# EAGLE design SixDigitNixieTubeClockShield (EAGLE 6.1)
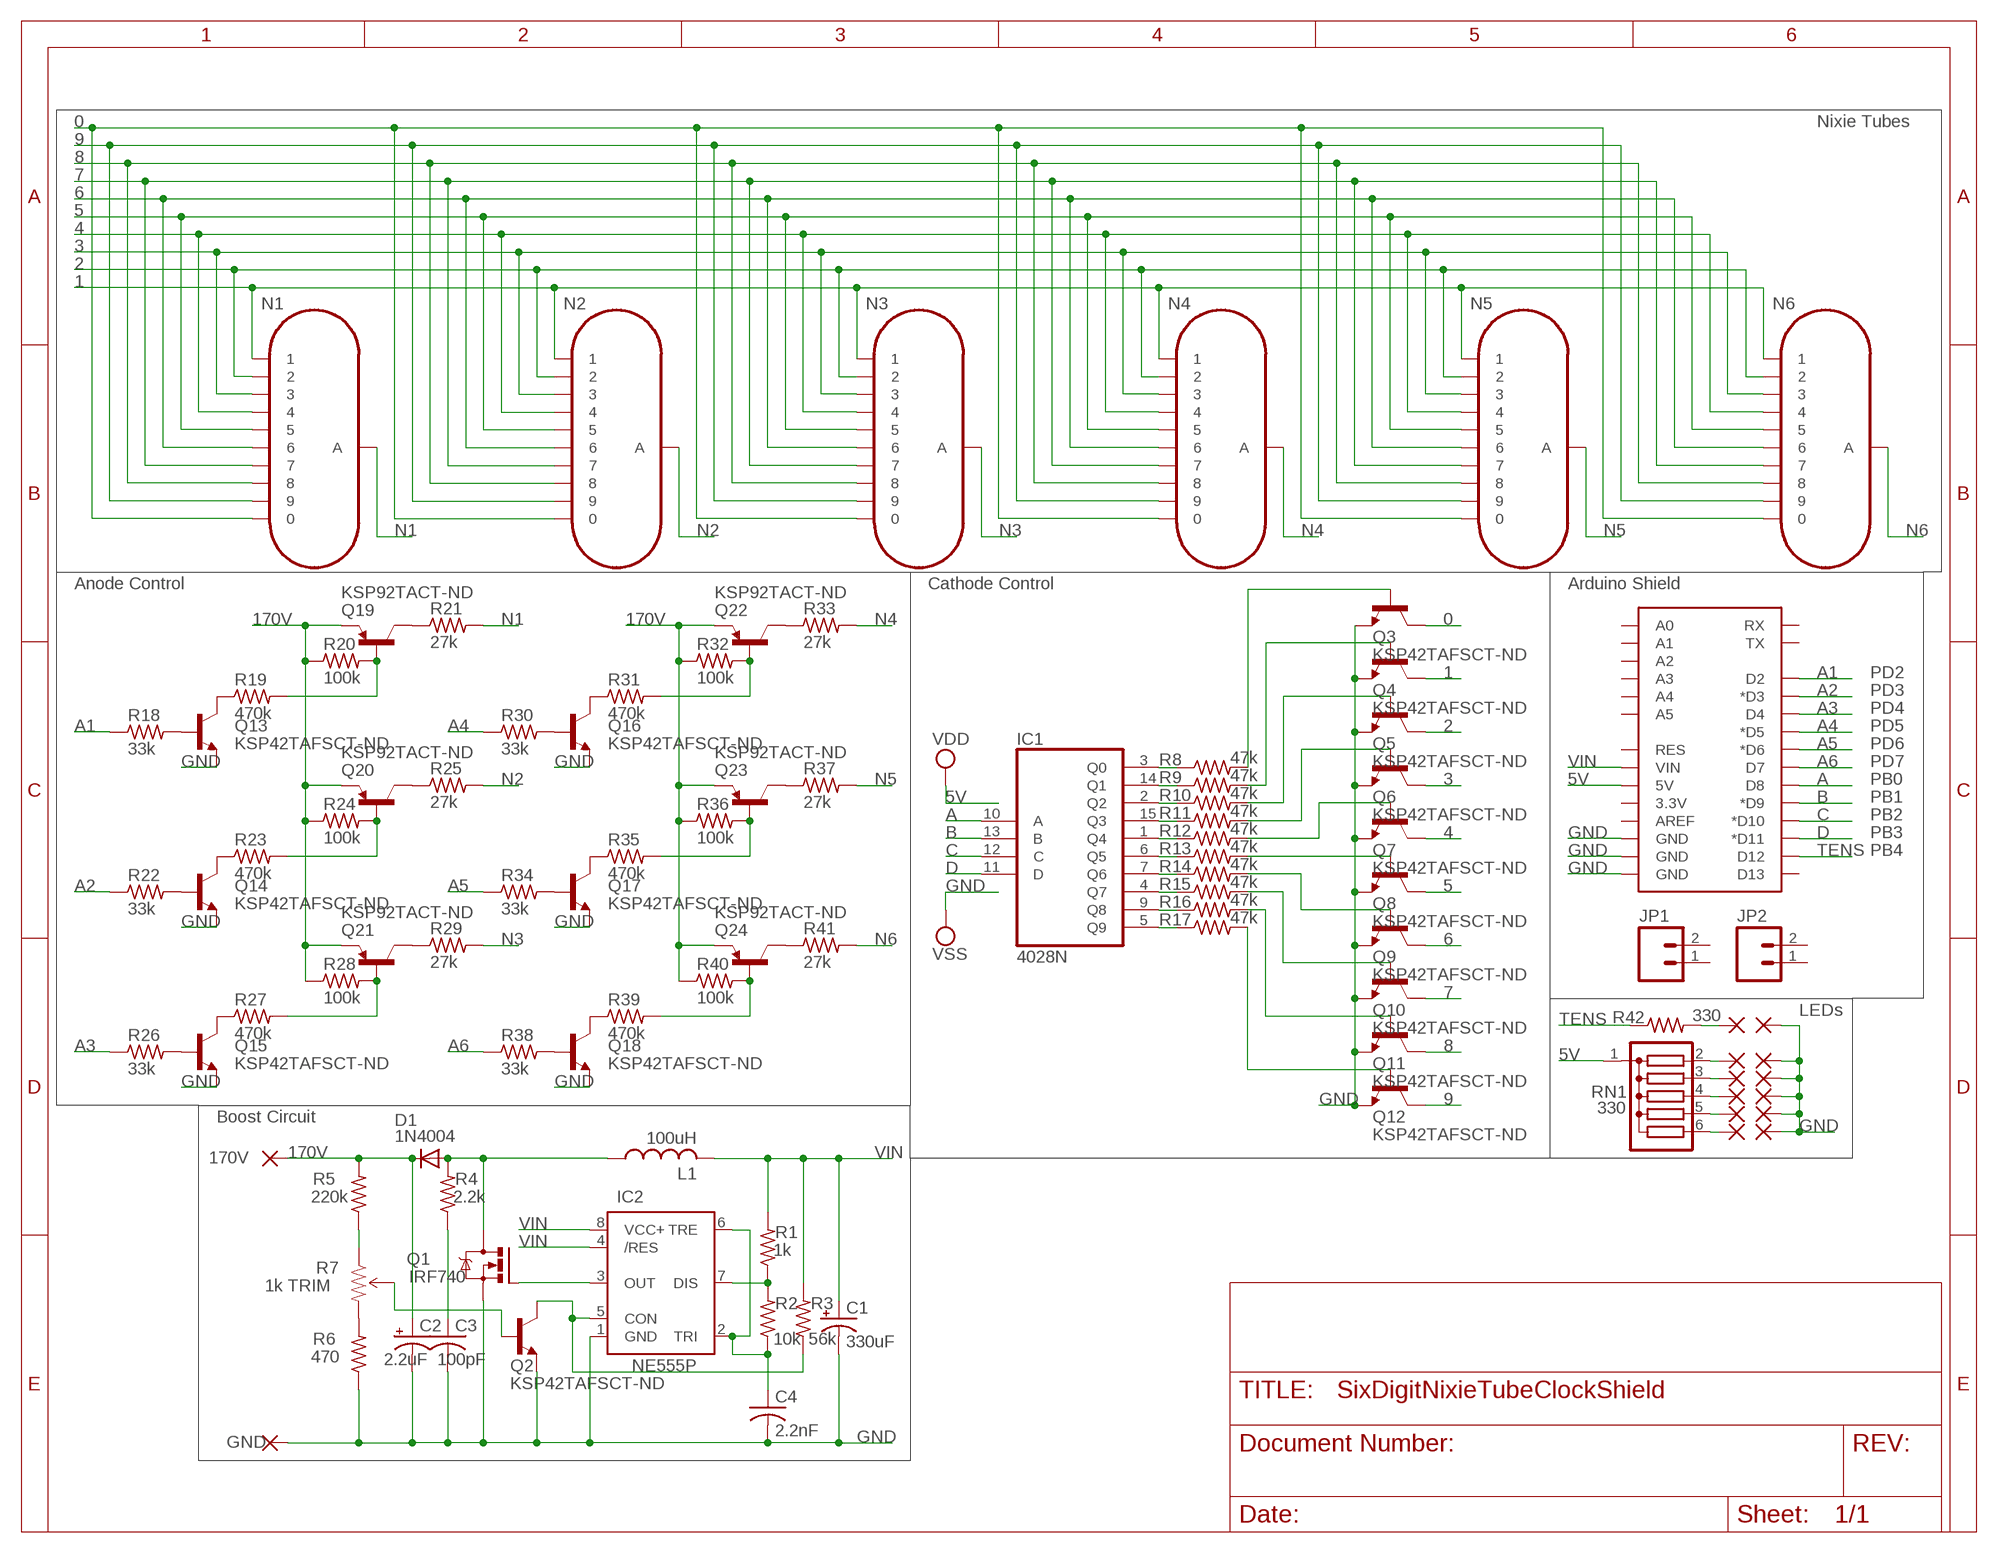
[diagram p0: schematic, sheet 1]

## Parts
C1  330uF  CPOL-USE2,5-6E  [E2,5-6E]
C2  2.2uF  CPOL-USE2,5-6E  [E2,5-6E]
C3  100pF  C-US050-025X075  [C050-025X075]
C4  2.2nF  C-US025-025X050  [C025-025X050]
D1  1N4004  [DO41-10]
IC1  4028N  [DIL16]
IC2  NE555P  [DIL-08]
JP1  M02PTH  [1X02]
JP2  M02PTH  [1X02]
L1  100uH  L-US6000-XXX-RC  [6000-XXXX-RC]
N1  IN-17  [IN-17]
N2  IN-17  [IN-17]
N3  IN-17  [IN-17]
N4  IN-17  [IN-17]
N5  IN-17  [IN-17]
N6  IN-17  [IN-17]
PAD1  1,6/0,8  [1,6/0,8]
PAD2  1,6/0,8  [1,6/0,8]
PAD3  1,6/0,8  [1,6/0,8]
PAD4  1,6/0,8  [1,6/0,8]
PAD5  1,6/0,8  [1,6/0,8]
PAD6  1,6/0,8  [1,6/0,8]
PAD7  1,6/0,8  [1,6/0,8]
PAD8  1,6/0,8  [1,6/0,8]
PAD9  1,6/0,8  [1,6/0,8]
PAD10  1,6/0,8  [1,6/0,8]
PAD11  1,6/0,8  [1,6/0,8]
PAD12  1,6/0,8  [1,6/0,8]
PAD13  GND  1,6/0,8  [1,6/0,8]
PAD14  170V  1,6/0,8  [1,6/0,8]
Q1  IRF740  [TO220BV]
Q2  KSP42TAFSCT-ND  TRANSISTOR_NPNTO-92-AMMO  [TO-92-AMMO]
Q3  KSP42TAFSCT-ND  TRANSISTOR_NPNTO-92-AMMO  [TO-92-AMMO]
Q4  KSP42TAFSCT-ND  TRANSISTOR_NPNTO-92-AMMO  [TO-92-AMMO]
Q5  KSP42TAFSCT-ND  TRANSISTOR_NPNTO-92-AMMO  [TO-92-AMMO]
Q6  KSP42TAFSCT-ND  TRANSISTOR_NPNTO-92-AMMO  [TO-92-AMMO]
Q7  KSP42TAFSCT-ND  TRANSISTOR_NPNTO-92-AMMO  [TO-92-AMMO]
Q8  KSP42TAFSCT-ND  TRANSISTOR_NPNTO-92-AMMO  [TO-92-AMMO]
Q9  KSP42TAFSCT-ND  TRANSISTOR_NPNTO-92-AMMO  [TO-92-AMMO]
Q10  KSP42TAFSCT-ND  TRANSISTOR_NPNTO-92-AMMO  [TO-92-AMMO]
Q11  KSP42TAFSCT-ND  TRANSISTOR_NPNTO-92-AMMO  [TO-92-AMMO]
Q12  KSP42TAFSCT-ND  TRANSISTOR_NPNTO-92-AMMO  [TO-92-AMMO]
Q13  KSP42TAFSCT-ND  TRANSISTOR_NPNTO-92-AMMO  [TO-92-AMMO]
Q14  KSP42TAFSCT-ND  TRANSISTOR_NPNTO-92-AMMO  [TO-92-AMMO]
Q15  KSP42TAFSCT-ND  TRANSISTOR_NPNTO-92-AMMO  [TO-92-AMMO]
Q16  KSP42TAFSCT-ND  TRANSISTOR_NPNTO-92-AMMO  [TO-92-AMMO]
Q17  KSP42TAFSCT-ND  TRANSISTOR_NPNTO-92-AMMO  [TO-92-AMMO]
Q18  KSP42TAFSCT-ND  TRANSISTOR_NPNTO-92-AMMO  [TO-92-AMMO]
Q19  KSP92TACT-ND  TRANSISTOR_PNP  [TO-92-AMMO]
Q20  KSP92TACT-ND  TRANSISTOR_PNP  [TO-92-AMMO]
Q21  KSP92TACT-ND  TRANSISTOR_PNP  [TO-92-AMMO]
Q22  KSP92TACT-ND  TRANSISTOR_PNP  [TO-92-AMMO]
Q23  KSP92TACT-ND  TRANSISTOR_PNP  [TO-92-AMMO]
Q24  KSP92TACT-ND  TRANSISTOR_PNP  [TO-92-AMMO]
R1  1k  R-US_0204/5  [0204/5]
R2  10k  R-US_0204/5  [0204/5]
R3  56k  R-US_0204/5  [0204/5]
R4  2.2k  R-US_0204/5  [0204/5]
R5  220k  R-US_0204/5  [0204/5]
R6  470  R-US_0204/5  [0204/5]
R7  1k TRIM  TRIMPOTPTH  [TRIM_POT_PTH]
R8  47k  R-US_0204/5  [0204/5]
R9  47k  R-US_0204/5  [0204/5]
R10  47k  R-US_0204/5  [0204/5]
R11  47k  R-US_0204/5  [0204/5]
R12  47k  R-US_0204/5  [0204/5]
R13  47k  R-US_0204/5  [0204/5]
R14  47k  R-US_0204/5  [0204/5]
R15  47k  R-US_0204/5  [0204/5]
R16  47k  R-US_0204/5  [0204/5]
R17  47k  R-US_0204/5  [0204/5]
R18  33k  R-US_0204/5  [0204/5]
R19  470k  R-US_0204/5  [0204/5]
R20  100k  R-US_0204/5  [0204/5]
R21  27k  R-US_0204/5  [0204/5]
R22  33k  R-US_0204/5  [0204/5]
R23  470k  R-US_0204/5  [0204/5]
R24  100k  R-US_0204/5  [0204/5]
R25  27k  R-US_0204/5  [0204/5]
R26  33k  R-US_0204/5  [0204/5]
R27  470k  R-US_0204/5  [0204/5]
R28  100k  R-US_0204/5  [0204/5]
R29  27k  R-US_0204/5  [0204/5]
R30  33k  R-US_0204/5  [0204/5]
R31  470k  R-US_0204/5  [0204/5]
R32  100k  R-US_0204/5  [0204/5]
R33  27k  R-US_0204/5  [0204/5]
R34  33k  R-US_0204/5  [0204/5]
R35  470k  R-US_0204/5  [0204/5]
R36  100k  R-US_0204/5  [0204/5]
R37  27k  R-US_0204/5  [0204/5]
R38  33k  R-US_0204/5  [0204/5]
R39  470k  R-US_0204/5  [0204/5]
R40  100k  R-US_0204/5  [0204/5]
R41  27k  R-US_0204/5  [0204/5]
R42  330  R-US_0204/5  [0204/5]
RN1  330  G05R  [SIL6]
U1  ARDUINO_SHIELDNO_SILK  [DUEMILANOVE_VIAS]

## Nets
0: N1.0 N2.0 N3.0 N4.0 N5.0 N6.0 Q3.3(C)
1: N1.1 N2.1 N3.1 N4.1 N5.1 N6.1 Q4.3(C)
2: N1.2 N2.2 N3.2 N4.2 N5.2 N6.2 Q5.3(C)
3: N1.3 N2.3 N3.3 N4.3 N5.3 N6.3 Q6.3(C)
4: N1.4 N2.4 N3.4 N4.4 N5.4 N6.4 Q7.3(C)
5: N1.5 N2.5 N3.5 N4.5 N5.5 N6.5 Q8.3(C)
5V: RN1.1 U1.5V ; supply symbol labelled VDD
6: N1.6 N2.6 N3.6 N4.6 N5.6 N6.6 Q9.3(C)
7: N1.7 N2.7 N3.7 N4.7 N5.7 N6.7 Q10.3(C)
8: N1.8 N2.8 N3.8 N4.8 N5.8 N6.8 Q11.3(C)
9: N1.9 N2.9 N3.9 N4.9 N5.9 N6.9 Q12.3(C)
170V: C2.+ D1.C PAD14.1(P) Q19.1(E) Q20.1(E) Q21.1(E) Q22.1(E) Q23.1(E) Q24.1(E) R5.2 R20.1 R24.1 R28.1 R32.1 R36.1 R40.1
A: IC1.10(A) U1.D8
A1: R18.1 U1.D2
A2: R22.1 U1.D3(*D3)
A3: R26.1 U1.D4
A4: R30.1 U1.D5(*D5)
A5: R34.1 U1.D6(*D6)
A6: R38.1 U1.D7
B: IC1.13(B) U1.D9(*D9)
C: IC1.12(C) U1.D10(*D10)
D: IC1.11(D) U1.D11(*D11)
GND: C1.- C2.- C3.2 C4.2 IC2.1(GND) PAD7.1(P) PAD8.1(P) PAD9.1(P) PAD10.1(P) PAD11.1(P) PAD12.1(P) PAD13.1(P) Q1.S Q2.1(E) Q3.1(E) Q4.1(E) Q5.1(E) Q6.1(E) Q7.1(E) Q8.1(E) Q9.1(E) Q10.1(E) Q11.1(E) Q12.1(E) Q13.1(E) Q14.1(E) Q15.1(E) Q16.1(E) Q17.1(E) Q18.1(E) R6.1 U1.GND@0(GND) U1.GND@1(GND) U1.GND@2(GND) ; supply symbol labelled VSS
N1: N1.A R21.2
N2: N2.A R25.2
N3: N3.A R29.2
N4: N4.A R33.2
N5: N5.A R37.2
N6: N6.A R41.2
N$1: IC2.3(OUT) Q1.G
N$2: IC2.7(DIS) R1.1 R2.2
N$3: C4.1 IC2.2(TRI) IC2.6(TRE) R2.1
N$4: IC2.5(CON) Q2.3(C) R3.1
N$5: C3.1 R4.1
N$6: D1.A L1.1 Q1.D R4.2
N$7: Q13.2(B) R18.2
N$8: R6.2 R7.3(CW)
N$9: R5.1 R7.1(CCW)
N$10: Q2.2(B) R7.2(WIPER)
N$11: IC1.3(Q0) R8.1
N$12: IC1.14(Q1) R9.1
N$13: IC1.2(Q2) R10.1
N$14: IC1.15(Q3) R11.1
N$15: IC1.1(Q4) R12.1
N$16: IC1.6(Q5) R13.1
N$17: IC1.7(Q6) R14.1
N$18: IC1.4(Q7) R15.1
N$19: IC1.9(Q8) R16.1
N$20: Q13.3(C) R19.1
N$21: IC1.5(Q9) R17.1
N$22: Q3.2(B) R8.2
N$23: Q4.2(B) R9.2
N$24: Q5.2(B) R10.2
N$25: Q6.2(B) R11.2
N$26: Q12.2(B) R17.2
N$27: Q19.3(C) R21.1
N$28: Q19.2(B) R19.2 R20.2
N$29: Q10.2(B) R15.2
N$30: Q9.2(B) R14.2
N$31: Q8.2(B) R13.2
N$32: Q14.2(B) R22.2
N$33: Q14.3(C) R23.1
N$34: Q20.3(C) R25.1
N$35: Q20.2(B) R23.2 R24.2
N$36: Q15.2(B) R26.2
N$37: Q15.3(C) R27.1
N$38: Q21.3(C) R29.1
N$39: Q21.2(B) R27.2 R28.2
N$40: Q16.2(B) R30.2
N$41: Q16.3(C) R31.1
N$42: Q22.3(C) R33.1
N$43: Q22.2(B) R31.2 R32.2
N$44: Q17.2(B) R34.2
N$45: Q17.3(C) R35.1
N$46: Q23.3(C) R37.1
N$47: Q23.2(B) R35.2 R36.2
N$48: Q18.2(B) R38.2
N$49: Q18.3(C) R39.1
N$50: Q24.3(C) R41.1
N$51: Q24.2(B) R39.2 R40.2
N$52: PAD1.1(P) R42.2
N$53: PAD2.1(P) RN1.2
N$54: PAD3.1(P) RN1.3
N$55: Q11.2(B) R16.2
N$56: Q7.2(B) R12.2
N$57: PAD4.1(P) RN1.4
N$58: PAD5.1(P) RN1.5
N$59: PAD6.1(P) RN1.6
TENS: R42.1 U1.D12
VIN: C1.+ IC2.4(/RES) IC2.8(VCC+) L1.2 R1.2 R3.2 U1.VIN
Unconnected: JP1.1 JP1.2 JP2.1 JP2.2 U1.3.3V U1.A0 U1.A1 U1.A2 U1.A3 U1.A4 U1.A5 U1.AREF U1.D13 U1.RES U1.RX U1.TX

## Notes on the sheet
- Nixie Tubes
- Anode Control | Cathode Control | Arduino Shield
- PD2
- PD3
- PD4
- PD5
- PD6
- PD7
- PB0
- PB1
- PB2
- PB3
- PB4
- LEDs
- Boost Circuit

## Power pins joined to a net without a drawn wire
5V: IC1.16(VDD)
GND: IC1.8(VSS)

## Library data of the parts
C1 C2 = resistor:CPOL-US: POLARIZED CAPACITOR, American symbol
C3 = rcl:C-US: CAPACITOR, American symbol
C4 = resistor:C-US: CAPACITOR, American symbol
D1 = diode:1N4004: DIODE
IC1 = 40xx:4028: BCD to decimal DECODER
IC2 = SparkFun-AnalogIC:NE555: General purpose bipolar Timer; MF: Arrow Electronics; MPN: NE555N; OC_FARNELL: 1467742; OC_NEWARK: 89K1486
JP1 JP2 = SparkFun-Connectors:M02: Header 2
L1 = rcl:L-US: INDUCTOR, American symbol
N1-N6 = russian-nixies:IN-17: IN-17: tiny numeric topview nixie tube
PAD1-PAD14 = wirepad:1,6/0,8: THROUGH-HOLE PAD
Q1 = transistor-power:IRF740: N-CHANNEL MOS FET
Q2-Q18 = SparkFun-DiscreteSemi:TRANSISTOR_NPN: Generic NPN BJT. MMBT2222 is the common NPN we use. Double check against datasheet- not all devices are the same!
Q19-Q24 = SparkFun-DiscreteSemi_tyler:TRANSISTOR_PNP: Generic PNP BJT. Double check pinouts against datasheets- not all devices are the same!
R1-R6 R8-R42 = resistor:R-US_: RESISTOR, American symbol
R7 = SparkFun-Electromechanical:TRIMPOT: Various small potentiometers for "set-and-forget" applications
RN1 = resistor-sil:G05R: SIL RESISTOR; OC_FARNELL: unknown; OC_NEWARK: unknown
U1 = SparkFun-Boards:ARDUINO_SHIELD: Arduino shield footprint

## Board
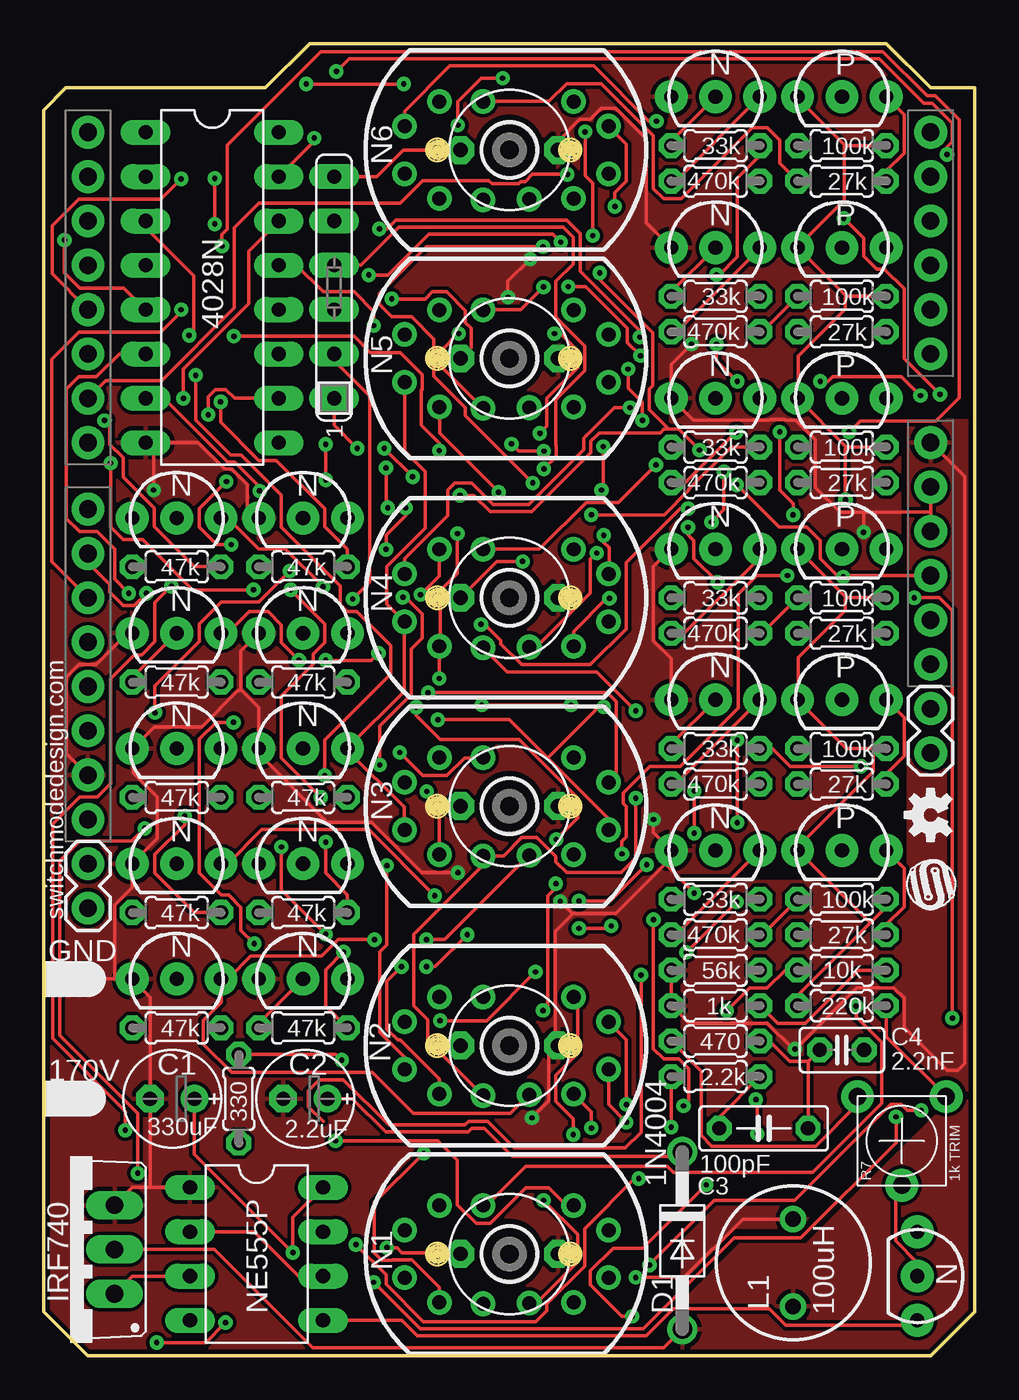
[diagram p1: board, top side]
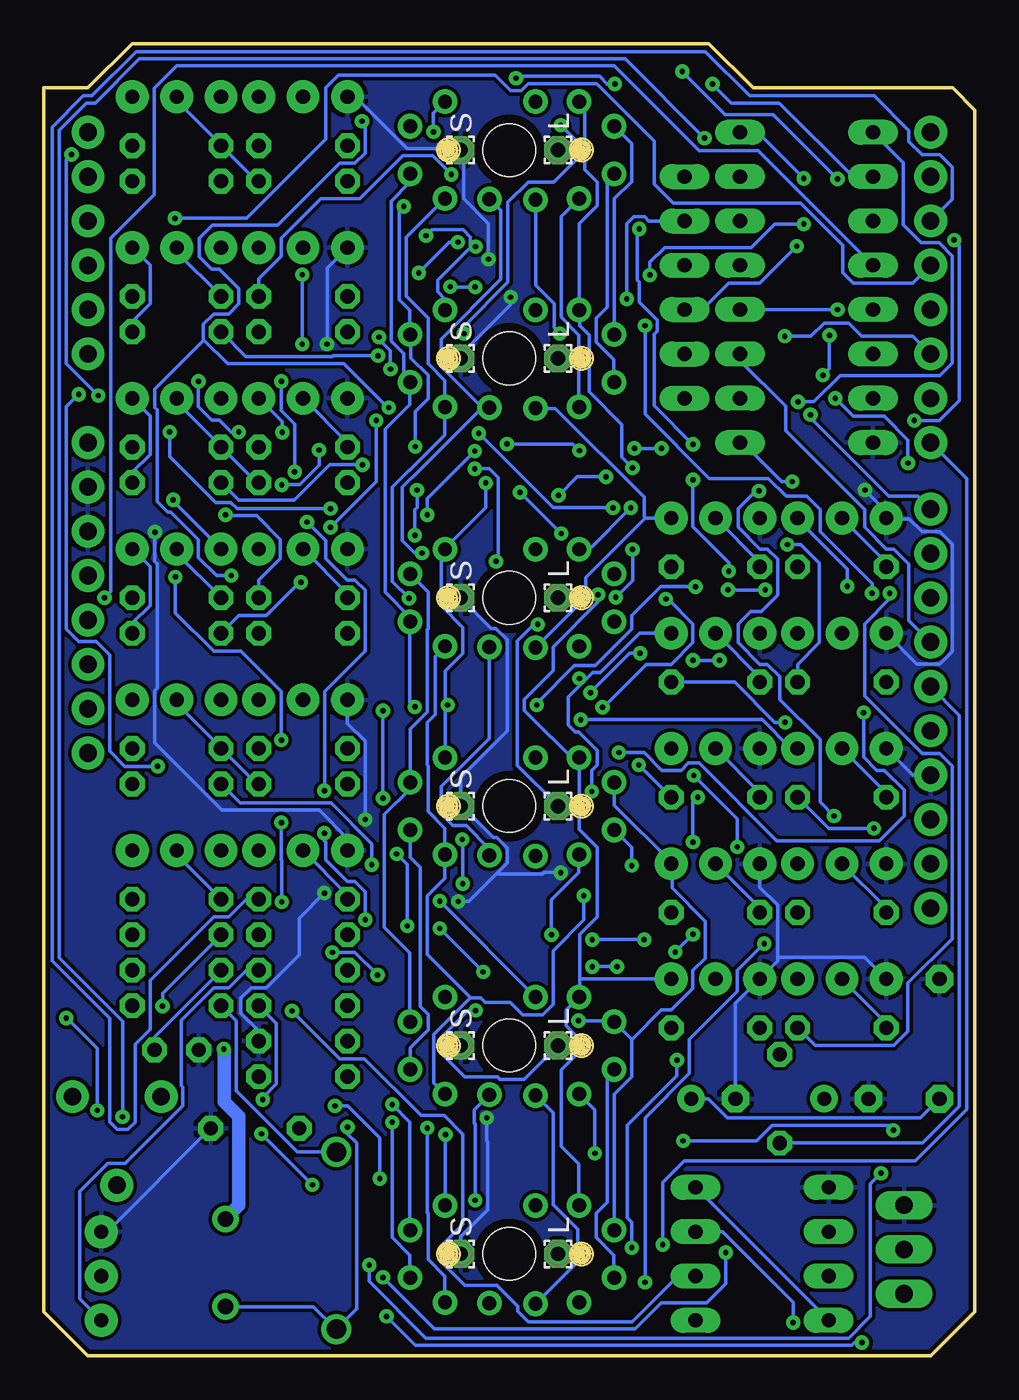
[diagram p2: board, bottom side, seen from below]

Size 53.34 x 75.18 mm. Coordinates in mm from the lower left corner, seen from the top.
Outline: 0,2.54 0,71.37 1.27,72.64 12.7,72.64 15.24,75.18 48.26,75.18 50.8,72.64 53.34,72.64 53.34,2.54 50.8,0 2.54,0 0,2.54
Copper layers (1*16): Top 0.035mm / dielectric 1.5mm / Bottom 0.035mm
Design rules: minimum track width 8mil, minimum drill 12mil, track to track 8mil, track to pad 8mil, pad to pad 8mil, via to via 8mil, smd to smd 8mil, copper to edge 10mil, drill to drill 6mil, minimum pad ring 12mil, minimum via ring 10mil, stop-mask expansion 4mil, vias tented up to drill 25mil, thermal gap 10mil
tRestrict: area 67.2,22.1 to 74.7,25.7
bRestrict: area 67.2,22.1 to 74.7,25.7

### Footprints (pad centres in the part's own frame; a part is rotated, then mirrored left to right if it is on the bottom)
E2,5-6E = drill 0.813 pad 1.575: + -1.27,0 | drill 0.813 pad 1.575 octagon: - 1.27,0
C050-025X075 = drill 0.813 octagon: 1 -2.54,0; 2 2.54,0
C025-025X050 = drill 0.813 octagon: 1 -1.27,0; 2 1.27,0
DO41-10 = drill 1.118: A 5.08,0; C -5.08,0
DIL16 = drill 0.813 long: 1 -8.89,-3.81; 2 -6.35,-3.81; 3 -3.81,-3.81; 4 -1.27,-3.81; 5 1.27,-3.81; 6 3.81,-3.81; 7 6.35,-3.81; 8 8.89,-3.81; 9 8.89,3.81; 10 6.35,3.81; 11 3.81,3.81; 12 1.27,3.81; 13 -1.27,3.81; 14 -3.81,3.81; 15 -6.35,3.81; 16 -8.89,3.81
DIL-08 = drill 0.813 long: 1 -3.81,-3.81; 2 -1.27,-3.81; 3 1.27,-3.81; 4 3.81,-3.81; 5 3.81,3.81; 6 1.27,3.81; 7 -1.27,3.81; 8 -3.81,3.81
1X02 = drill 1.016 pad 1.88: 1 0,0; 2 2.54,0
6000-XXXX-RC = drill 0.9 pad 1.422: 1 -2.5,0; 2 2.5,0
IN-17 = drill 0.8: 0 2.777,4; 1 1.365,6; 2 -1.365,6; 3 -2.778,4; 4 -2.858,1.5; 5 -2.818,-1.143; 6 -2.778,-3.683; 7 -1.365,-5.683; 8 1.365,-5.683; 9 2.777,-3.683; A 2.777,1.5
1,6/0,8 = drill 0.813 pad 1.6 octagon: 1 0,0
TO220BV = drill 1.016 long: D 0,-2.54; G -2.54,-2.54; S 2.54,-2.54
TO-92-AMMO = drill 0.813 pad 1.88: 1 -2.54,0; 2 0,0; 3 2.54,0
0204/5 = drill 0.813 octagon: 1 -2.54,0; 2 2.54,0
TRIM_POT_PTH = drill 1 pad 1.88: 1 -2.54,-2.54; 2 0,2.54; 3 2.54,-2.54
SIL6 = drill 0.813 long: 1 -6.35,0; 2 -3.81,0; 3 -1.27,0; 4 1.27,0; 5 3.81,0; 6 6.35,0
DUEMILANOVE_VIAS = drill 1.016 pad 1.88: 3.3V 50.8,13.97; 5V 50.8,16.51; A0 50.8,29.21; A1 50.8,31.75; A2 50.8,34.29; A3 50.8,36.83; A4 50.8,39.37; A5 50.8,41.91; AREF 2.54,2.54; D2 2.54,36.83; D3 2.54,34.29; D4 2.54,31.75; D5 2.54,29.21; D6 2.54,26.67; D7 2.54,24.13; D8 2.54,20.32; D9 2.54,17.78; D10 2.54,15.24; D11 2.54,12.7; D12 2.54,10.16; D13 2.54,7.62; GND@0 50.8,19.05; GND@1 50.8,21.59; GND@2 2.54,5.08; RES 50.8,11.43; RX 2.54,41.91; TX 2.54,39.37; VIN 50.8,24.13
3,0 = hole 3: 0,0

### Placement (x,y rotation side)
C1  7.37,14.73 180 top
C2  14.99,14.73 180 top
C3  41.24,13.03 0 top
C4  45.72,17.53 180 top
D1  36.58,6.6 270 top
IC1  9.65,61.21 270 top
IC2  12.19,5.84 270 top
JP1  2.54,28.19 270 top
JP2  50.8,37.08 270 top
L1  42.93,5.33 90 top
N1  26.67,5.84 90 top
N2  26.67,17.78 90 top
N3  26.67,31.5 90 top
N4  26.67,43.43 90 top
N5  26.67,57.15 90 top
N6  26.67,69.09 90 top
PAD1  23.88,5.84 0 bottom
PAD2  23.88,17.78 0 bottom
PAD3  23.88,31.5 0 bottom
PAD4  23.88,43.43 0 bottom
PAD5  23.88,57.15 0 bottom
PAD6  23.88,69.09 0 bottom
PAD7  29.46,5.84 0 bottom
PAD8  29.46,17.78 0 bottom
PAD9  29.46,31.5 0 bottom
PAD10  29.46,43.43 0 bottom
PAD11  29.46,57.15 0 bottom
PAD12  29.46,69.09 0 bottom
PAD13  2.03,21.59 0 top
PAD14  2.03,14.73 0 top
Q1  1.52,6.1 90 top
Q2  50.04,4.57 270 top
Q3  14.86,21.59 0 top
Q4  14.86,28.19 0 top
Q5  14.86,34.8 0 top
Q6  14.86,41.4 0 top
Q7  14.86,48.01 0 top
Q8  7.62,21.59 0 top
Q9  7.62,28.19 0 top
Q10  7.62,34.8 0 top
Q11  7.62,41.4 0 top
Q12  7.62,48.01 0 top
Q13  38.48,28.96 0 top
Q14  38.48,37.59 0 top
Q15  38.48,46.23 0 top
Q16  38.48,54.86 0 top
Q17  38.48,63.5 0 top
Q18  38.48,72.14 0 top
Q19  45.72,28.96 0 top
Q20  45.72,37.59 0 top
Q21  45.72,46.23 0 top
Q22  45.72,54.86 0 top
Q23  45.72,63.5 0 top
Q24  45.72,72.14 0 top
R1  38.48,20.07 180 top
R2  45.72,22.1 0 top
R3  38.48,22.1 180 top
R4  38.48,16 180 top
R5  45.72,20.07 180 top
R6  38.48,18.03 180 top
R7  49.15,12.32 180 top
R8  14.86,18.8 180 top
R9  14.86,25.4 180 top
R10  14.86,32 180 top
R11  14.86,38.61 180 top
R12  14.86,45.21 180 top
R13  7.62,18.8 180 top
R14  7.62,25.4 180 top
R15  7.62,32 180 top
R16  7.62,38.61 180 top
R17  7.62,45.21 180 top
R18  38.48,26.16 180 top
R19  38.48,24.13 0 top
R20  45.72,26.16 180 top
R21  45.72,24.13 180 top
R22  38.48,34.8 180 top
R23  38.48,32.77 0 top
R24  45.72,34.8 180 top
R25  45.72,32.77 180 top
R26  38.48,43.43 180 top
R27  38.48,41.4 0 top
R28  45.72,43.43 180 top
R29  45.72,41.4 180 top
R30  38.48,52.07 180 top
R31  38.48,50.04 0 top
R32  45.72,52.07 180 top
R33  45.72,50.04 180 top
R34  38.48,60.71 180 top
R35  38.48,58.67 0 top
R36  45.72,60.71 180 top
R37  45.72,58.67 180 top
R38  38.48,69.34 180 top
R39  38.48,67.31 0 top
R40  45.72,69.34 180 top
R41  45.72,67.31 180 top
R42  11.18,14.73 90 top
RN1  16.64,61.21 90 top
U1  0,28.19 0 top
U$1  [3,0]  26.67,5.84 0 top
U$2  [3,0]  26.67,17.78 0 top
U$3  [3,0]  26.67,31.5 0 top
U$4  [3,0]  26.67,43.43 0 top
U$5  [3,0]  26.67,57.15 0 top
U$6  [3,0]  26.67,69.09 0 top
U$7  [OSHW-LOGO-S]  50.8,30.99 90 top
U$8  [SWITCHMODE_LOGO_S]  52.45,25.4 90 top

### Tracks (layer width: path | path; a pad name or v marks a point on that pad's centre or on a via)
0  (via drill 0.3)
  Top 0.203: v21.59,43.61 22.66,44.68 22.66,46.2 N4.0 | v19.61,50.88 19.61,48.69 v19.71,48.59
  Bottom 0.203: N6.0 22.66,71.86 22.35,71.55 22.35,67.97 21.64,67.26 21.64,65.89 22.66,64.87 22.66,59.94 N5.0 22.63,59.84 22.63,59.03 22.1,58.5 22.1,55.24 20.22,53.37 20.22,51.49 v19.61,50.88 | N1.0 22.68,8.64 22.68,11 23.7,12.01 23.7,16.38 22.76,17.32 22.76,18.24 23.42,18.9 23.42,19.81 22.68,20.55 N2.0 22.63,20.65 22.63,21.59 | 22.63,21.59 22.63,24.16 21.64,25.15 21.64,29.13 22.66,30.15 22.66,34.27 N3.0 22.73,33.91 25.81,36.98 25.81,37.62 24.16,39.27 24.16,40.62 21.59,43.18 v21.59,43.61 | 22.63,21.59 Q3.3 | v19.71,48.59 22.07,46.23 22.66,46.23 N4.0
1  (via drill 0.3)
  Top 0.203: v33.58,54.33 32.69,54.33 30.94,52.58 30.94,51.92 27.79,48.77 25.76,48.77 24.51,50.01 23.55,50.01 23.14,49.61 23.14,48.13 20.68,45.67 N4.1 | v35.1,70.74 34.67,70.74 31.5,73.91 23.27,73.91 20.68,71.32 N6.1 | v22.71,19.2 25.38,19.2 v28.17,22 | v30.66,24.49 32.36,24.49 v32.51,24.64 | v33.12,28.75 33.12,29.46 33.38,29.72 33.38,31.47 33.2,31.65 33.2,32.26 34.72,33.78 36.45,33.78 39.78,37.11 39.78,43.64 40.84,44.7 v42.6,44.7
  Bottom 0.203: N3.1 20.65,32.84 20.65,31.55 17.4,28.3 Q4.3 17.35,28.12 17.35,26.8 15.44,24.89 15.44,22.78 16.15,22.07 16.15,21.06 17.4,19.81 17.96,19.81 19.58,18.19 19.66,18.14 | 19.66,18.14 19.66,15.98 20.65,14.99 20.65,7.21 N1.1 | 19.66,18.14 20.65,19.13 N2.1 20.75,19.2 v22.71,19.2 | v33.58,54.33 33.63,54.33 36.14,56.84 42.8,56.84 44.16,58.2 | 44.16,58.2 44.2,58.24 44.2,59.11 43.61,59.69 42.75,59.69 42.16,60.27 42.16,61.14 43.28,62.26 43.71,62.26 44.42,62.97 44.42,64.03 43.69,64.77 39.93,64.77 36.37,68.33 35.51,68.33 34.92,68.91 34.92,70.56 v35.1,70.74 | N5.1 20.65,58.52 20.65,66.29 19.66,67.28 19.66,69.44 20.65,70.43 N6.1 | v30.66,24.49 v28.17,22 | v32.51,24.64 32.51,28.14 v33.12,28.75 | v42.6,44.7 43.43,44.7 44.48,45.74 44.48,46.76 46.05,48.34 46.23,48.34 46.84,48.95 46.84,54.2 46.97,54.33 46.97,55.4 44.16,58.2
2  (via drill 0.3)
  Top 0.203: N3.2 20.65,30.15 20.65,31.45 17.4,34.7 Q5.3 17.45,34.87 20.65,38.08 20.65,42.06 N4.2 20.6,42.14 19.66,43.08 19.66,45.24 21.84,47.42 21.84,50.67 20.68,51.84 N5.2 | v19.66,28.09 19.66,23.55 19.25,23.14 19.25,18.54 20.65,17.14 20.65,16.43 N2.2
  Bottom 0.203: N5.2 20.68,55.8 20.68,57.07 21.69,58.09 21.69,59.46 21.06,60.1 21.06,67.33 N6.2 | N1.2 20.68,4.5 20.68,5.77 21.69,6.78 21.69,8.15 21.06,8.79 21.06,16.03 N2.2 | v19.66,28.09 19.66,29.13 20.65,30.12 N3.2
3  (via drill 0.3)
  Top 0.203: v21.77,11.61 18.95,8.79 18.95,5.89 19.36,5.49 19.96,5.49 19.99,5.51 21.08,5.51 22.66,3.94 22.66,3.07 N1.3 | v21.95,32.33 22.66,31.62 22.66,28.73 N3.3 | v22.66,38.81 22.66,40.64 N4.3 22.71,40.74 22.71,43.84 23.7,44.83 v23.7,47.12 | v26.06,49.48 22.68,52.86 22.68,54.36 N5.3 | v20.5,22.3 19.66,21.46 19.66,18.72 20.27,18.11 20.42,18.11 22.66,15.88 22.66,15.01 N2.3 | v21.92,22.3 22.43,22.3 v24.26,24.13
  Bottom 0.203: v21.77,11.61 21.77,14.1 22.66,14.99 N2.3 | N5.3 22.68,54.38 22.68,58.5 23.7,59.51 23.7,65.28 22.68,66.29 N6.3 | v21.95,32.33 21.95,33.55 21.64,33.86 21.64,34.7 22.68,35.74 22.89,35.74 23.29,36.14 23.29,37.74 22.44,38.59 | 22.44,38.59 21.89,39.14 21.46,39.14 19.2,41.4 Q6.3 | 22.44,38.59 v22.66,38.81 | v23.7,47.12 v26.06,49.48 | v21.92,22.3 v20.5,22.3 | v24.26,24.13 24.26,26.14 22.68,27.71 22.68,28.7 N3.3
4  (via drill 0.3)
  Top 0.203: N2.4 25.15,14.94 22,18.09 22,19.25 21.21,20.04 21.21,24.16 25.15,28.09 25.15,28.63 N3.4 25.27,28.65 26.34,28.65 27.38,29.69 28.25,29.69 29.34,28.6 29.34,28.3 29.95,27.69 33.07,27.69 33.91,28.52 v33.91,31.95 | v23.77,58.57 23.72,58.57 22.76,57.61 22.76,56.69 25.15,54.3 N5.4 | v33.91,36.96 31.67,39.19 26.54,39.19 25.17,40.56 N4.4
  Bottom 0.203: N1.4 25.15,3 22.76,5.38 22.76,7.26 24.16,8.66 24.16,13.92 25.15,14.91 N2.4 | 18.9,48.01 22.3,44.6 22.3,43.43 25.15,40.59 N4.4 | Q7.3 18.9,48.01 | N5.4 25.15,54.28 24.03,54.28 18.95,49.2 18.95,48.08 18.9,48.01 | v23.77,58.57 24.11,58.9 24.11,60.3 25.15,61.34 25.15,66.22 N6.4 | v33.91,36.96 v33.91,31.95
5  (via drill 0.3)
  Top 0.203: v28.63,8.91 30.58,6.96 30.58,5.38 28.25,3.05 27.81,3.05 N1.5 | N2.5 27.79,14.96 26.72,13.89 21.16,13.89 18.82,16.23 10.77,16.23 9.14,17.86 9.14,19.23 10.16,20.24 Q8.3 10.24,21.64 10.59,21.64 11.86,22.91 15.93,22.91 16.87,23.85 v18.95,23.85 | v31.67,46 31.32,45.64 31.32,43.71 28.25,40.64 27.81,40.64 N4.5 | v21.92,23.85 22.96,23.85 27.79,28.68 N3.5
  Bottom 0.203: v28.63,8.91 28.63,13.28 28.68,13.34 28.68,14.1 N2.5 | N3.5 27.81,28.7 27.81,29.06 29.13,30.38 29.92,30.38 30.58,31.04 30.58,32.61 27.81,35.38 N4.5 | N6.5 27.79,66.27 27.15,65.63 27.15,61.7 30.58,58.27 30.58,56.69 28.25,54.36 27.81,54.36 N5.5 28.27,54.28 32.23,50.32 32.26,50.32 32.79,49.78 32.79,46.71 32.08,46 v31.67,46 | v21.92,23.85 v18.95,23.85
5V  (via drill 0.3)
  Top 0.203: RN1.1 16.64,53.31 v17.96,51.99 | v21.13,50.37 v19.51,51.99 | v23.85,49.3 24.64,49.3 25.58,48.36 27.96,48.36 31.34,51.74 31.34,52.4 31.83,52.88 35.31,52.88 35.51,53.09 35.74,53.09 | 35.74,53.09 36.37,53.09 v37.57,51.89 | v39.7,49.91 42.14,47.47 43.71,47.47 44.48,46.71 44.48,45.7 45.47,44.7 45.8,44.7 | U1.5V 45.8,44.7 | v9.8,64.85 v9.8,67.46 | v18.62,61.92 19.71,61.92 22.05,64.26 29.16,64.26 v29.62,63.8 | v31.85,62.05 31.85,61.67 34.9,58.62 34.9,55.6 34.7,55.4 34.7,54.2 35.74,53.16 35.74,53.09 | 16,13.44 15.16,14.28 15.16,15.19 15.8,15.82 17.17,15.82 19.76,13.23 24.13,13.23 24.33,13.44 25.43,13.44 26.95,11.91 33.33,11.91 34.21,12.8 v34.21,21.82 | v39.7,26.01 v36.8,23.11 | v39.73,35.28 v39.73,30.56 | v45.8,44.63 45.8,44.7
  Bottom 0.203: v19.51,51.99 v17.96,51.99 | v21.13,50.37 22.78,50.37 v23.85,49.3 | v37.57,51.89 37.57,51.03 38.68,49.91 v39.7,49.91 | IC1.16 12.45,70.1 v9.8,67.46 | v9.8,64.85 11.48,64.85 12.83,63.5 17.78,63.5 18.62,62.66 v18.62,61.92 | v29.62,63.8 30.1,63.8 v31.85,62.05 | v34.21,21.82 35.51,23.11 v36.8,23.11 | v39.7,26.01 39.7,28.4 39.73,28.42 v39.73,30.56 | v39.73,35.28 39.73,38.08 42.04,40.39 43.61,40.39 45.8,42.57 v45.8,44.63
6  (via drill 0.3)
  Top 0.203: v31.37,13.06 31.37,13.97 30.35,14.99 N2.6 | Q9.3 10.54,28.19 12.5,30.15 18.62,30.15 v22.4,26.36 | v32.41,43.41 32.26,43.41 30.35,41.5 N4.6
  Bottom 0.203: N6.6 30.35,66.29 32.56,64.08 32.56,60.71 31.32,59.46 31.32,56.84 30.35,55.88 30.35,54.38 N5.6 30.38,54.28 30.38,52.76 32.41,50.72 32.44,50.72 33.38,49.78 33.38,44.37 v32.41,43.41 | N4.6 30.35,40.64 30.91,40.08 30.91,36.75 31.37,36.3 31.37,33.86 31.32,33.81 31.32,31.19 30.35,30.23 N3.6 30.38,28.63 30.38,27.36 31.37,26.36 31.37,23.01 28.93,20.57 28.91,20.5 | v31.37,13.06 31.37,8.2 31.32,8.15 31.32,5.54 30.35,4.57 30.35,3.07 N1.6 | v22.4,26.36 22.4,24.97 24.16,23.22 24.16,20.14 24.77,19.53 25.91,19.53 26.62,20.24 28.04,20.24 28.3,20.5 28.91,20.5 | 28.91,20.5 30.99,18.41 30.99,15.65 N2.6
7  (via drill 0.3)
  Top 0.203: v33.38,13.39 32.36,14.4 N2.7 | v22.58,36.45 26.67,36.45 28.87,34.25 | 28.87,34.25 32.33,30.79 32.33,30.15 N3.7 | v32.08,37.19 31.8,37.19 28.87,34.25
  Bottom 0.203: N6.7 32.36,67.23 33.43,66.17 33.43,58.14 32.72,57.43 32.72,56.21 32.38,55.88 N5.7 32.36,54.51 33.78,53.09 33.78,43.76 32.36,42.34 32.36,42.09 N4.7 32.36,41.96 32.36,37.47 v32.08,37.19 | v33.38,13.39 33.38,6.78 32.36,5.77 32.36,4.5 N1.7 | N3.7 32.33,30.12 32.33,28.55 31.77,27.99 31.77,20.02 31.32,19.56 31.32,18.67 32.33,17.65 32.33,16.43 N2.7 | Q10.3 10.54,34.8 12.19,36.45 v22.58,36.45
8  (via drill 0.3)
  Top 0.203: v32.72,65.86 32.72,66.65 33.38,67.31 33.38,69.42 32.36,70.43 N6.8 | v33.38,14.4 33.38,18.11 32.36,19.13 N2.8 | Q11.3 10.54,41.4 11.79,42.65 12.85,42.65 13.61,41.88 13.61,40.87 v14.63,39.85 | v16.15,39.85 18.77,39.85 v19.18,40.26 | v22.02,38 32.28,38 32.79,37.49 32.79,33.3 N3.8 | v32.05,52.09 32.05,49.71 v31.95,49.61 | v32.08,47.02 32.08,46.61 32.38,46.3 32.38,44.83 N4.8
  Bottom 0.203: v32.72,65.86 32.97,65.61 32.97,60.53 32.36,59.92 32.36,58.52 N5.8 32.31,58.42 32.31,57.17 31.32,56.19 31.32,54.84 32.05,54.1 v32.05,52.09 | v33.38,14.4 32.36,13.39 N1.8 | N4.8 32.33,44.78 31.32,43.76 31.32,41.66 31.37,41.6 31.37,36.88 32.33,35.92 32.33,32.87 N3.8 32.38,32.77 32.38,32.46 33.83,31.01 33.83,24.56 32.36,23.09 32.36,19.15 N2.8 | v16.15,39.85 v14.63,39.85 | v19.18,40.26 19.76,40.26 v22.02,38 | v31.95,49.61 31.95,48.62 32.08,48.49 v32.08,47.02
9  (via drill 0.3)
  Top 0.203: v31.45,64.19 31.45,67.18 31.01,67.61 v31.01,70.13 | v30.33,12.68 30.33,13.59 29.34,14.58 29.34,16.08 30.58,17.32 30.58,20.32 30.35,20.55 N2.9 | Q12.3 10.54,48.01 12.32,46.23 13.84,46.23 v16,44.07 | v30.2,37.29 v25.09,37.29 | v16.71,12.32 22.58,12.32 23.7,11.2 23.7,8.66 24.77,7.59 25.58,7.59 27.61,9.63 28.93,9.63 29.92,8.64 30.33,8.64 N1.9 | v4.67,12.93 4.67,14.02 0.51,18.19 0.51,30.48 2.06,32.03 3.07,32.03 3.83,32.79 3.83,38.81 5.18,40.16 5.61,40.16 6.38,40.92 6.38,43.16 v7.32,44.09 | v28.6,63.55 21.92,63.55 19.23,60.86 19.23,60.25 19.94,59.54 21.08,59.54 22.35,58.27 22.35,56.13 24.16,54.33 24.16,53.87 v28.02,50.01
  Bottom 0.203: 28.91,63.5 30.76,61.65 30.76,60.96 30.35,60.55 30.35,59.94 N5.9 | 28.91,63.5 28.91,64.11 29.31,64.52 31.11,64.52 v31.45,64.19 | v31.01,70.13 31.01,71.2 30.35,71.86 N6.9 | v30.33,12.68 30.33,8.64 N1.9 | 30.33,37.29 30.33,39.24 29.34,40.23 29.34,41.73 30.58,42.98 30.58,45.97 N4.9 30.3,46.3 28.02,48.59 v28.02,50.01 | 30.33,37.29 30.33,34.29 N3.9 | v16,44.07 18.01,44.07 19.66,42.42 19.66,41.63 21.74,39.55 22.94,39.55 25.09,37.39 v25.09,37.29 | v30.2,37.29 30.33,37.29 | v16.71,12.32 12.5,12.32 11.61,13.21 4.95,13.21 v4.67,12.93 | v7.32,44.09 7.32,45.09 10.16,47.93 Q12.3 | v28.6,63.55 28.83,63.55 28.91,63.5
170V  (via drill 0.3)
  Top 0.203: 45.9,69.34 R40.1 | 45.9,69.34 43.18,72.06 Q24.1 | 45.97,52.07 R32.1 | 45.97,52.07 Q22.1 43.23,54.94 43.23,57.28 45.92,59.97 45.92,60.63 45.97,60.71 | 45.97,60.71 R36.1 | 45.97,60.71 Q23.1 43.2,63.58 45.85,66.22 45.85,69.27 45.9,69.34 | 47.52,34.8 45.97,34.8 Q20.1 43.23,37.67 43.23,40.01 45.92,42.7 45.92,43.36 45.97,43.43 | 47.52,34.8 R24.1 | 45.97,43.43 R28.1 | Q21.1 45.97,43.43 | R5.2 43.18,20.65 47.33,24.8 | 47.33,24.8 48.26,25.73 R20.1 | 47.33,24.8 Q19.1 43.23,29.03 43.23,29.18 47.52,33.48 47.52,34.8 | C2.+ 17.68,14.73 19.58,12.83 24.31,12.83 24.51,13.03 25.25,13.03 26.85,11.43 36.32,11.43 D1.C | v45.92,49.05 45.92,51.99 45.97,52.07
  Bottom 0.203: C2.+ 15.27,14.73 14.17,13.64 3.12,13.64 PAD14.1 | D1.C 38.81,11.68 42.32,15.19 42.32,19.2 R5.2 | v45.92,49.05 45.92,48.97 Q21.1
A  (via drill 0.3)
  Top 0.203: IC1.10 10.95,54.86 10.44,55.37 9.83,55.37 9.42,54.97 v9.42,53.92
  Bottom 0.203: v9.42,53.92 9.42,53.75 4.93,49.25 3.28,49.25 U1.D8
A1
  Bottom 0.203: R18.1 41.73,26.16 42.75,25.15 43.61,25.15 47.24,21.51 47.24,18.72 48.11,17.86 48.11,13.39 48.51,12.98 49.12,12.98 49.55,13.41 49.55,19.33 52.86,22.63 52.86,70.41 51.08,72.19 50.57,72.19 48.03,74.73 15.44,74.73 12.9,72.19 5.77,72.19 3.79,70.21 3.79,69.57 3.02,68.81 2.01,68.81 1.29,68.1 1.29,66.27 U1.D2
A2  (via drill 0.3)
  Top 0.203: R22.1 41.73,34.8 42.75,33.78 v46.81,33.78 | v51.33,55.09 49.28,57.15 49.28,61.14 48.16,62.26 47.73,62.26 46.97,63.02 46.97,64.03 v45.82,65.18
  Bottom 0.203: v46.81,33.78 48.69,33.78 49.55,34.65 49.55,40.16 50.32,40.92 51.33,40.92 52.05,41.63 52.05,54.38 v51.33,55.09 | v45.82,65.18 41.71,65.18 37.19,69.7 37.19,72.67 36.47,73.38 27.48,73.38 26.59,72.49 25.98,72.49 25.58,72.9 21.67,72.9 18.36,69.6 18.36,67.13 17.27,66.04 9.98,66.04 7.57,63.63 7.57,62.05 6.99,61.47 3.56,61.47 U1.D3
A3  (via drill 0.3)
  Top 0.203: v42.93,48.18 42.93,48.84 42.16,49.61 v42.16,52.93 | v44.48,55.83 44.91,55.83 45.19,56.11 49.12,56.11 v50.22,55.02 | v51.74,68.83 51.74,69.27 52.05,69.57 52.05,70.64 50.9,71.78 50.39,71.78 47.85,74.32 17.5,74.32 v16.76,73.58 | v7.87,67.44 6.71,66.27 2.01,66.27 0.48,64.75 0.48,62 U1.D4
  Bottom 0.203: R26.1 41.02,44.45 39.78,45.7 39.78,46.76 41.15,48.13 42.88,48.13 v42.93,48.18 | v42.16,52.93 42.6,52.93 43.28,53.62 43.71,53.62 44.48,54.38 v44.48,55.83 | v50.22,55.02 52.05,56.84 52.05,68.53 v51.74,68.83 | v16.76,73.58 14.3,71.12 11.56,71.12 v7.87,67.44
A4  (via drill 0.3)
  Top 0.203: R30.1 39.37,52.07 36.96,49.66 36.96,49.61 35.53,48.18 v31.37,48.18 | v28.65,51.84 27.2,51.84 v26.8,52.25 | v22.66,51.87 22.66,52.3 21.64,53.31 21.64,55.32 21.69,55.37 21.69,56.21 20.42,57.48 18.72,57.48 17.78,58.42 v10.9,58.42
  Bottom 0.203: v31.37,48.18 31.37,49.12 v28.65,51.84 | v26.8,52.25 23.04,52.25 v22.66,51.87 | v10.9,58.42 9.4,58.42 8.64,59.18 7.24,59.18 6.48,58.42 3.56,58.42 U1.D5
A5  (via drill 0.3)
  Top 0.203: v30,67.69 27.99,67.69 27.58,67.28 27.33,67.28 27.2,67.16 25.68,67.16 25.5,67.33 21.72,67.33 20.42,66.04 12.32,66.04 10.92,64.64 10.92,60.05 6.76,55.88 3.56,55.88 U1.D6
  Bottom 0.203: R34.1 41.02,61.72 39.73,63.02 39.73,64.03 37.47,66.29 35.23,66.29 32.77,68.76 31.06,68.76 v30,67.69
A6  (via drill 0.3)
  Top 0.203: R38.1 41.02,68.76 39.73,67.46 39.73,62.97 38.71,61.95 v38.53,61.95 | v38.53,57.96 38.53,57.02 v39.73,55.83 | v38.96,50.65 38.96,48.49 v38.25,47.78 | v37.26,29.95 v37.26,32.38 | v34.92,24.99 34.92,17.6 35.51,17.02 36.37,17.02 36.96,16.43 36.96,14.63 v36.65,14.33 | v34.09,10.16 33.86,10.16 30.99,7.29 30.99,5.13 28.83,2.97 28.83,2.59 28.19,1.96 21.74,1.96 19.61,4.09 19.61,4.65 v17.88,6.38
  Bottom 0.203: v38.53,57.96 v38.53,61.95 | v39.73,55.83 39.73,54.15 38.96,53.39 v38.96,50.65 | v38.25,47.78 37.19,46.71 37.19,45.7 35.94,44.45 35.51,44.45 34.92,43.87 34.92,40.39 37.24,38.08 37.24,32.41 v37.26,32.38 | v37.26,29.95 37.26,29.52 37.19,29.44 37.19,28.42 35.94,27.18 35.51,27.18 34.92,26.59 v34.92,24.99 | v36.65,14.33 35.92,14.33 34.09,12.5 v34.09,10.16 | v17.88,6.38 17.88,9.93 16.64,11.18 3.43,11.18 0.48,14.12 0.48,50.27 U1.D7
B  (via drill 0.3)
  Top 0.203: IC1.13 14.48,62.48 16,60.96 17.78,60.96 18.9,59.84 v18.9,59.03 | v5.89,43.69 5.18,42.98 4.57,42.98 3.79,43.76 3.79,44.2 2.54,45.44 U1.D9
  Bottom 0.203: v18.9,59.03 18.9,53.95 15.21,50.27 11.84,50.27 10.82,49.25 9.63,49.25 8.87,48.49 8.87,47.22 5.89,44.25 v5.89,43.69
C  (via drill 0.3)
  Top 0.203: v7.87,59.94 7.87,59.82 6.71,58.65 2.01,58.65 0.46,57.1 0.46,45.52 U1.D10
  Bottom 0.203: v7.87,59.94 IC1.12
D
  Bottom 0.203: IC1.11 13.46,57.02 10.85,54.41 10.85,53.01 6.33,48.49 6.33,47.47 5.08,46.23 4.65,46.23 3.79,45.36 3.79,42.14 U1.D11
GND  (via drill 0.3)
  Top 0.203: Q7.1 11.66,48.67 11.66,49.91 10.77,50.8 10.36,50.8 8.84,52.32 IC1.8 6.3,52.25 v6.3,49.61 | 11.3,38.18 12.32,37.16 Q5.1 12.37,34.72 12.37,34.44 16.26,30.56 18.8,30.56 21.67,27.69 v23.72,27.69 | 11.3,38.18 11.3,40.39 Q6.1 | Q11.1 4.83,41.4 3.02,39.6 2.01,39.6 1.29,38.89 1.29,34.52 U1.GND@2 | 11.3,38.18 11.23,38.12 11.12,38.12 9.04,36.04 6.33,36.04 Q10.1 5.13,34.72 5.13,33.4 6.5,32.03 6.5,29.64 5.13,28.27 Q9.1 5.08,26.85 4.06,25.83 4.06,21.59 | 6.1,9.65 5.08,9.65 Q1.S | 6.1,9.65 IC2.1 | 6.1,9.65 C1.- 6.1,20.55 5.13,21.51 Q8.1 4.06,21.59 | 4.06,21.59 PAD13.1 | v26.59,60.66 26.59,61.57 v27.86,62.84 | U1.GND@1 50.8,48.34 | 50.8,48.34 U1.GND@0 | v37.11,57.96 35.94,56.79 Q16.1 36.02,54.81 37.21,53.62 41.55,53.62 41.58,53.65 42.47,53.65 42.49,53.62 43.08,53.62 44.2,52.5 44.2,49.76 45.62,48.34 46.97,48.34 | 46.97,48.34 50.8,48.34 | PAD12.1 29.46,69.6 30.71,70.84 31.29,70.84 31.93,71.48 32.77,71.48 34.52,69.72 34.52,64.92 Q17.1 | 43.79,16.87 43.79,13.06 C3.2 | C4.2 43.79,16.87 | R6.1 41.55,18.03 42.72,16.87 43.79,16.87 | Q14.1 35.94,39.95 34.92,40.97 34.92,45.21 Q15.1 | v27.96,13.64 28.93,14.61 28.93,17.25 PAD8.1 29.31,17.75 29.31,24.31 30.32,25.31 | Q13.1 35.94,28.52 32.77,25.35 30.35,25.35 30.32,25.31 | v34.92,30.73 34.92,30 35.89,29.03 Q13.1 | 30.32,25.31 v29.59,26.04 | v37.26,26.52 35.66,28.12 Q13.1 | v46.97,47.19 46.97,48.34
  Bottom 0.203: v6.3,49.61 5.08,48.39 Q12.1 5,47.95 3.76,47.95 3.02,47.22 2.01,47.22 1.29,46.51 1.29,40.36 2.01,39.65 3.33,39.65 Q11.1 | U1.GND@2 3.56,33.27 Q10.1 | C2.- 13.72,20.19 Q3.1 12.27,21.67 11.3,22.63 11.3,22.84 | Q4.1 12.32,26.85 11.3,25.83 11.3,22.84 | 11.3,22.84 6.33,22.84 Q8.1 | PAD11.1 29.46,57.35 26.59,60.22 v26.59,60.66 | v27.86,62.84 27.86,64.87 29.29,66.29 29.29,68.91 PAD12.1 29.52,69.16 32.51,69.16 35.48,72.14 Q18.1 | v37.11,57.96 37.11,62.33 Q17.1 | Q2.1 49.71,7.11 C3.2 | PAD10.1 27.71,41.68 27.43,41.68 26.8,41.05 26.8,35.81 29.46,33.15 PAD9.1 29.39,31.45 29.34,31.45 27.58,29.69 27.38,29.69 26.8,29.11 26.8,28.25 27.37,27.67 | PAD7.1 29.46,6.83 27.91,8.38 27.91,12.27 27.96,12.32 v27.96,13.64 | Q14.1 35.94,36.25 34.92,35.23 v34.92,30.73 | 27.37,27.67 29.01,26.04 v29.59,26.04 | R6.1 41.02,18.62 42.04,19.63 42.04,20.5 41.45,21.08 40.59,21.08 38.71,22.96 38.71,25.07 v37.26,26.52 | v46.97,47.19 46.97,45.52 46.84,45.39 46.84,38.25 46.97,38.12 46.97,35.1 43.13,31.27 37.57,31.27 35.94,29.64 Q13.1 | v23.72,27.69 24.69,27.69 24.77,27.61 27.3,27.61 27.37,27.67
  pour Bottom (isolate 0.203): 2.54,0 50.8,0 53.34,2.54 53.34,72.64 50.8,72.64 48.26,75.18 15.24,75.18 12.7,72.64 1.27,72.64 0,71.37 0,2.54
  pour Top (isolate 0.203): 2.54,0 36.07,0 36.07,27.69 49.02,27.69 49.02,54.1 53.34,54.1 53.34,72.64 50.8,72.64 48.26,75.18 15.24,75.18 12.7,72.64 1.27,72.64 0,71.37 0,2.54
N1  (via drill 0.3)
  Top 0.203: v46.53,20.04 46.53,19.43 48.01,17.96 48.01,14.48 44.04,10.52 36.07,10.52 35.71,10.87 27.61,10.87 25.38,8.64 25.17,8.64 N1.A
  Bottom 0.203: v46.53,20.04 46.53,20.78 R21.2
N2  (via drill 0.3)
  Top 0.203: v30.66,26.06 32.46,26.06 v34.54,28.14
  Bottom 0.203: v30.66,26.06 25.17,20.57 N2.A | v34.54,28.14 34.54,29.34 36.88,31.67 42.09,31.67 R25.2
N3  (via drill 0.3)
  Top 0.203: v20.4,34.57 21.72,33.25 23.09,33.25 24.11,34.27 25.15,34.27 N3.A | v6.38,36.85 6.38,38.38 8.91,40.92 8.91,41.94 10.16,43.18 12.32,43.18 v14.1,44.96 | v16.15,52.22 v16.15,50.19 | v19.23,64.57 19.66,64.57 20.17,65.08 29.95,65.08 30.73,64.29 30.73,62.15 34.14,58.75 v34.14,58.37 | v33.48,56.54 33.48,55.45 34.29,54.63 v34.29,53.59 | v36.91,47.47 36.91,47.04 37.24,46.71 37.24,45.7 v38.61,44.32
  Bottom 0.203: v20.4,34.57 18.95,34.57 17.93,33.55 16.82,33.55 16.41,33.96 15.8,33.96 11.35,29.52 5.49,29.52 4.06,30.94 4.06,32.44 5.18,33.55 5.61,33.55 6.38,34.31 v6.38,36.85 | v14.1,44.96 14.1,45.47 16.15,47.52 v16.15,50.19 | v16.15,52.22 18.36,54.43 18.36,58.55 18.19,58.73 18.19,59.33 19.23,60.38 19.23,61.52 19.33,61.62 19.33,64.47 v19.23,64.57 | v34.14,58.37 34.14,58.27 33.48,57.61 v33.48,56.54 | v34.29,53.59 34.29,50.09 v36.91,47.47 | v38.61,44.32 38.68,44.32 40.59,42.42 42.16,42.42 R29.2
N4  (via drill 0.3)
  Top 0.203: v35.08,51.05 32.92,48.9 31.06,48.9 28.4,46.23 25.17,46.23 N4.A
  Bottom 0.203: v35.08,51.05 36.96,51.05 38.99,49.02 42.16,49.02 R33.2
N5  (via drill 0.3)
  Top 0.203: v28.63,61.24 27.33,59.94 25.17,59.94 N5.A | v30.05,61.27 31.04,61.27 33.43,58.88 33.43,58.06 v34.19,57.3
  Bottom 0.203: v28.63,61.24 30.02,61.24 v30.05,61.27 | v34.19,57.3 36.75,57.3 36.8,57.25 41.76,57.25 R37.2
N6
  Top 0.203: R41.2 42.16,68.33 42.16,69.65 41.45,70.36 40.59,70.36 36.52,66.29 35.51,66.29 34.92,66.88 34.92,69.9 31.93,72.9 29.95,72.9 28.93,71.88 25.17,71.88 N6.A
N$1
  Top 0.203: IC2.3 5.08,4.57 Q1.G
N$2  (via drill 0.3)
  Top 0.203: v10.41,1.91 9.27,0.76 v6.48,0.76 | v33.71,2.26 33.12,2.26 31.32,4.06 31.32,4.88 32.61,6.17 34.31,6.17 v37.95,9.8 | v40.87,12.72 40.87,14.61 v40.79,14.68 | R2.2 46.66,22.1 43.61,19.05 42.04,19.05 R1.1
  Bottom 0.203: IC2.7 14.45,7.11 10.41,3.07 v10.41,1.91 | v6.48,0.76 6.91,0.76 7.06,0.61 32.05,0.61 v33.71,2.26 | v40.87,12.72 v37.95,9.8 | v40.79,14.68 40.79,14.78 40.01,15.57 40.01,19.05 R1.1
N$3  (via drill 0.3)
  Top 0.203: IC2.2 12.06,7.11 14.61,4.57 IC2.6 | R2.1 42.47,22.1 41.45,21.08 40.44,21.08 v39.12,19.76
  Bottom 0.203: C4.1 46.99,18.29 R2.1 | v39.12,19.76 36.37,17.02 34.98,17.02 31.73,13.77 30.4,13.77 29.34,12.7 29.34,7.54 30.58,6.3 30.58,5.38 29.23,4.04 27.38,4.04 26.19,2.85 26.19,2.56 25.58,1.96 19.63,1.96 17.02,4.57 IC2.6
N$4
  Top 0.203: IC2.5 20.5,2.03 21.39,1.14 34.52,1.14 36.07,2.69 41.55,2.69 42.49,1.75 49.76,1.75 Q2.3
  Bottom 0.203: R3.1 41.73,22.1 42.75,21.08 43.61,21.08 45.47,19.23 45.47,15.49 45.36,15.39 45.36,14.33 48.67,11.02 49.68,11.02 51.28,9.42 51.28,3.28 Q2.3
N$5
  Top 0.203: R4.1 38.71,13.69 38.71,13.06 C3.1
N$6  (via drill 0.3)
  Top 0.203: v35.94,13.11 R4.2 | Q1.D 9.78,6.1 15.42,0.46 35.51,0.46 D1.A
  Bottom 0.203: v35.94,13.11 35.94,12.72 35.41,12.19 35.41,2.69 D1.A 36.65,1.57 37.9,2.82 42.93,2.82 L1.1
  pour Top (isolate 0.203): 36.58,0 50.8,0 53.34,2.54 53.34,14.73 52.07,14.73 43.69,6.35 39.88,6.35 36.58,3.05
N$7
  Bottom 0.203: R18.2 35.94,26.42 Q13.2
N$8
  Top 0.203: R6.2 37.67,16.31 37.67,12.62 38.28,12.01 44.22,12.01 46.61,14.4 R7.3
N$9
  Top 0.203: R5.1 48.26,18.29 R7.1
N$10
  Top 0.203: Q2.2 50.04,5.33 48.79,6.58 48.79,9.42 R7.2
N$11  (via drill 0.3)
  Top 0.203: IC1.3 5.84,64.64 8.59,61.9 8.59,58.73 v8.33,58.47 | v8.71,56.19 8.71,53.62 10.72,51.61 11.33,51.61 13.61,49.33 13.61,47.47 16.99,44.09 16.99,43.05 17.4,42.65 17.93,42.65 19.89,40.69 19.89,39.06 16.1,35.28 v16.1,33.25 | v13.61,29.16 13.61,26.7 v16.15,24.16 | v17.17,23.14 16.15,22.12 16.15,20.04 R8.1
  Bottom 0.203: v8.33,58.47 8.33,56.57 v8.71,56.19 | v16.1,33.25 13.61,30.76 v13.61,29.16 | v17.17,23.14 v16.15,24.16
N$12  (via drill 0.3)
  Top 0.203: R9.1 17.4,26.42 16.15,27.66 v16.15,29.44 | v15.88,32 13.61,34.27 13.61,37.82 15.44,39.65 15.44,40.21 16.1,40.87 16.1,41.94 v14.15,43.89 | v12.01,43.89 8.53,43.89 5.66,46.76 4.55,46.76 3.83,47.47 v3.83,51.16 | v8,54.86 8,56.54 11.73,60.27 11.73,63.3 IC1.14
  Bottom 0.203: v16.15,29.44 16.15,31.73 v15.88,32 | v12.01,43.89 v14.15,43.89 | v3.83,51.16 3.83,52.48 5.21,53.85 6.99,53.85 v8,54.86
N$13  (via drill 0.3)
  Top 0.203: v20.62,72.87 v15.04,72.87 | v26.29,73.2 25.07,73.2 23.72,71.86 v23.72,70.51 | v29.26,58.57 29.62,58.57 30.58,57.61 30.58,56.62 28.83,54.86 28.83,53.26 v28.42,52.86 | v20.73,48.59 20.73,48.16 19.61,47.04 v19.61,46.2 | v20.57,43.46 20.73,43.46 21.69,42.49 21.69,41.12 21.06,40.49 21.06,37.9 19.25,36.09 v19.25,33.86
  Bottom 0.203: IC1.2 6.99,67.56 11.2,71.78 13.95,71.78 v15.04,72.87 | v20.62,72.87 21.06,72.87 21.49,73.3 26.19,73.3 v26.29,73.2 | v23.72,70.51 22.76,69.55 22.76,68.63 24.13,67.26 25.58,67.26 26.75,66.09 26.75,61.52 29.26,59 v29.26,58.57 | v28.42,52.86 24.16,48.59 v20.73,48.59 | v19.61,46.2 19.61,44.42 v20.57,43.46 | R10.1 v19.25,33.86
N$14  (via drill 0.3)
  Top 0.203: v10.87,36.3 9.88,36.3 8.91,35.33 8.91,27.66 10.16,26.42 10.59,26.42 11.3,25.7 11.3,24.38 v12.06,23.62 | v18.9,4.22 21.57,1.55 34.34,1.55 39.55,6.76 43.36,6.76 48.82,12.22 v48.82,13.69 | v15.49,69.77 15.49,69.6 IC1.15
  Bottom 0.203: R11.1 13.77,38.61 11.46,36.3 v10.87,36.3 | v12.06,23.62 13.61,22.07 13.61,20.88 16.36,18.14 16.36,16.18 18.9,13.64 v18.9,4.22 | v48.82,13.69 48.82,19.18 52.45,22.81 52.45,70.23 50.9,71.78 50.39,71.78 47.85,74.32 20.04,74.32 v15.49,69.77
N$15  (via drill 0.3)
  Top 0.203: R12.1 17.4,46.23 16.1,47.52 16.1,48.54 13.34,51.31 12.32,51.31 10.13,53.49 v10.13,54.66
  Bottom 0.203: v10.13,54.66 9.22,54.66 7.72,56.16 2.01,56.16 1.29,56.87 1.29,63.02 2.06,63.78 3.07,63.78 4.12,64.82 4.12,68.38 IC1.1
N$16  (via drill 0.3)
  Top 0.203: IC1.6 4.32,57.4 3.02,56.11 2.01,56.11 1.29,55.4 1.29,47.98 2.06,47.22 3.07,47.22 4.06,46.23 4.06,44.5 v4.88,43.69
  Bottom 0.203: v4.88,43.69 4.88,43.38 6.33,41.94 6.33,37.82 3.02,34.52 2.01,34.52 1.29,33.81 1.29,23.9 3.83,21.36 3.83,18.59 4.65,17.78 9.14,17.78 R13.1
N$17  (via drill 0.3)
  Top 0.203: IC1.7 6.88,54.86 10.54,51.21 10.95,51.21 12.37,49.78 v12.37,49.55 | v8.08,30.94 8.08,30.43 6.38,28.73 6.38,27.66 8.64,25.4 R14.1
  Bottom 0.203: v12.37,49.55 12.55,49.55 13.56,48.54 13.56,47.47 12.32,46.23 11.89,46.23 11.3,45.64 11.3,43.59 12.24,42.65 12.85,42.65 13.56,41.94 13.56,40.87 12.32,39.62 11.89,39.62 11.18,38.91 11.18,37.62 8.87,35.31 8.87,31.73 v8.08,30.94
N$18  (via drill 0.3)
  Top 0.203: v49.86,43.43 51.31,43.43 52.05,42.7 v52.05,19.36 | v50.27,14.07 49.45,14.07 49.12,14.4 48.51,14.4 43.03,8.91 38.41,8.91 v34.7,5.21 | v5.38,10.46 5.38,13.89 0.91,18.36 0.91,28.35 2.06,29.49 5.05,29.49 v5.79,30.23
  Bottom 0.203: IC1.4 12.42,69.06 15.8,69.06 20.65,73.91 45.72,73.91 47.02,72.62 47.02,66.52 49.51,64.03 49.51,43.79 v49.86,43.43 | v52.05,19.36 52.05,19.41 50.27,17.63 v50.27,14.07 | v34.7,5.21 34.7,4.27 31.45,1.02 7.24,1.02 5.99,2.26 5.99,9.86 v5.38,10.46 | v5.79,30.23 8.38,30.23 R15.1
N$19  (via drill 0.3)
  Top 0.203: v10.74,46.48 9.91,46.48 8.91,47.47 8.91,48.54 v10.46,50.09
  Bottom 0.203: R16.1 10.16,39.62 8.91,40.87 8.91,45.41 9.98,46.48 v10.74,46.48 | v10.46,50.09 11.07,50.09 13.31,52.32 IC1.9
N$20
  Top 0.203: R19.1 36.2,24.13 Q13.3
N$21  (via drill 0.3)
  Top 0.203: R17.1 8.64,45.21 6.33,47.52 6.33,48.56 4.55,50.34 4.55,51.46 3.79,52.22 3.79,53.29 v3.48,53.59 | v1.19,63.93 1.19,62.05 2.06,61.19 4.6,61.19 IC1.5
  Bottom 0.203: v3.48,53.59 2.03,53.59 0.89,54.74 0.89,63.63 v1.19,63.93
N$22
  Top 0.203: R8.2 12.32,19.05 Q3.2
N$23
  Bottom 0.203: R9.2 12.32,25.65 Q4.2
N$24
  Bottom 0.203: R10.2 12.32,32.26 Q5.2
N$25
  Bottom 0.203: R11.2 12.32,38.86 Q6.2
N$26
  Bottom 0.203: R17.2 5.08,45.47 Q12.2
N$27
  Top 0.203: R21.1 48.26,24.71 49.28,25.73 49.28,27.94 Q19.3
N$28
  Top 0.203: R19.2 41.15,24.13 R20.2
  Bottom 0.203: Q19.2 45.72,28.7 R20.2
N$29
  Bottom 0.203: R15.2 5.08,32.26 Q10.2
N$30
  Bottom 0.203: R14.2 5.08,25.65 Q9.2
N$31
  Bottom 0.203: R13.2 5.08,19.05 Q8.2
N$32
  Top 0.203: R22.2 35.94,35.05 Q14.2
N$33
  Top 0.203: R23.1 36.2,32.77 Q14.3
N$34
  Top 0.203: R25.1 48.26,33.35 49.28,34.37 49.28,36.58 Q20.3
N$35
  Bottom 0.203: R23.2 41.15,32.77 R24.2 43.23,34.87 45.72,37.36 Q20.2
N$36
  Bottom 0.203: R26.2 35.94,43.69 Q15.2
N$37
  Top 0.203: R27.1 36.7,41.4 41.02,45.72 Q15.3
N$38
  Bottom 0.203: R29.1 48.26,41.99 47.24,43 47.24,45.21 Q21.3
N$39
  Top 0.203: R27.2 41.15,41.4 R28.2
  Bottom 0.203: Q21.2 45.72,45.97 R28.2
N$40
  Bottom 0.203: R30.2 35.94,52.32 Q16.2
N$41  (via drill 0.3)
  Top 0.203: R31.1 36.75,50.04 39.62,52.91 v39.67,52.91
  Bottom 0.203: v39.67,52.91 39.67,53.52 Q16.3
N$42
  Bottom 0.203: R33.1 48.26,50.62 47.24,51.64 47.24,53.85 Q22.3
N$43
  Bottom 0.203: R31.2 41.15,50.04 R32.2 43.23,52.15 45.72,54.63 Q22.2
N$44
  Top 0.203: R34.2 35.94,60.96 Q17.2
N$45
  Top 0.203: R35.1 36.27,58.67 41.02,63.42 Q17.3
N$46
  Bottom 0.203: R37.1 48.26,59.26 47.24,60.27 47.24,62.48 Q23.3
N$47
  Top 0.203: R35.2 41.15,58.67 R36.2
  Bottom 0.203: Q23.2 45.72,63.25 R36.2
N$48
  Top 0.203: R38.2 35.94,69.6 Q18.2
N$49
  Top 0.203: R39.1 36.2,67.31 Q18.3
N$50
  Top 0.203: R41.1 48.26,67.89 49.28,68.91 49.28,71.12 Q24.3
N$51
  Bottom 0.203: R39.2 41.15,67.31 R40.2 43.23,69.42 45.72,71.91 Q24.2
N$52  (via drill 0.3)
  Top 0.203: R42.2 16.74,17.27 v17.07,16.94 | v19.66,6.2 20.24,6.2 20.52,5.92 23.8,5.92 PAD1.1
  Bottom 0.203: v17.07,16.94 17.07,16.05 19.91,13.21 19.91,7.9 19.66,7.64 v19.66,6.2
N$53  (via drill 0.3)
  Top 0.203: RN1.2 16.64,57.02 18.67,54.99 18.67,44.32 v17.7,43.36 | v21.34,37.16 21.34,36.68 22.71,35.31 27.23,35.31 30.58,31.95 30.58,30.81 v29.36,29.59 | v29.34,27.05 29.34,26.8 28.88,26.34 28.88,20.07 v28.6,19.79
  Bottom 0.203: v17.7,43.36 17.58,43.36 16.15,41.94 16.15,40.87 17.4,39.62 18.82,39.62 21.29,37.16 v21.34,37.16 | v29.36,29.59 29.36,29.16 29.34,29.13 v29.34,27.05 | v28.6,19.79 29.03,19.79 30.58,18.24 30.58,17.32 29.23,15.98 27.33,15.98 27.2,15.85 25.81,15.85 PAD2.1
N$54  (via drill 0.3)
  Top 0.203: v10.21,63.58 10.21,64.24 10.52,64.54 10.52,69.37 15.88,74.73 48.06,74.73 50.6,72.19 51.08,72.19 52.45,70.81 52.45,54.91 51.1,53.57 46.76,53.57 v46.13,52.93 | v36.91,48.54 36.47,48.54 33.38,45.44 33.38,41.66 31.32,39.6 27.38,39.6 26.19,40.79 26.19,41 25.27,41.91 v25.04,41.91
  Bottom 0.203: RN1.3 15.62,59.94 14.1,61.47 12.32,61.47 v10.21,63.58 | v46.13,52.93 46.13,51.54 43.48,48.9 42.62,48.9 42.27,48.54 v36.91,48.54 | v25.04,41.91 25.27,41.91 26.21,40.97 26.21,33.83 PAD3.1
N$55
  Top 0.203: R16.2 5.08,38.86 Q11.2
N$56
  Bottom 0.203: R12.2 12.32,45.47 Q7.2
N$57  (via drill 0.3)
  Top 0.203: RN1.4 18.16,62.48 20.34,64.67 29.77,64.67 30.33,64.11 30.33,62.56 29.34,61.57 29.34,59.51 30.99,57.86 30.99,56.44 29.34,54.79 29.34,52.17 29.36,52.15 29.36,51.54 v28.65,50.83 | v27.43,45.52 25.96,45.52 PAD4.1
  Bottom 0.203: v28.65,50.83 27.81,50.83 27.3,50.32 27.3,45.64 v27.43,45.52
N$58  (via drill 0.3)
  Top 0.203: v19.94,60.55 21.84,60.55 22.25,60.96 23.09,60.96 24.16,59.89 24.16,59.21 24.49,58.88 24.49,57.76 PAD5.1
  Bottom 0.203: RN1.5 18.67,65.02 18.92,65.28 19.53,65.28 19.94,64.87 v19.94,60.55
N$59
  Top 0.203: RN1.6 19.07,67.56 20.6,69.09 PAD6.1
TENS
  Bottom 0.203: R42.1 3,12.19 0.89,14.3 0.89,36.7 U1.D12
VIN  (via drill 0.3)
  Top 0.203: R3.2 R1.2 36.02,20.02 36.98,19.05 41.45,19.05 42.93,17.58 v43.03,17.58 43.1,17.63 46.56,21.08 48.69,21.08 49.28,20.5 49.28,18.82 51.74,16.36 52.35,16.36 52.76,16.76 52.76,50.37 U1.VIN | C1.+ 8.64,11.56 v14.28,5.92 14.28,7.92 IC2.8 | v33.91,4.5 36.7,4.5 40.03,7.82 L1.2
  Bottom 0.203: 42.93,7.87 L1.2 | v14.28,5.92 14.28,4.14 15.37,3.05 17.96,3.05 19.46,1.55 30.96,1.55 v33.91,4.5 | IC2.8 IC2.4
  Bottom 0.762: 42.93,7.87 42.16,8.64 42.16,13.72 43,14.55 43,17.3 v43.03,17.58
  pour Top (isolate 0.203): 53.34,15.24 51.05,15.24 43.18,7.37 39.62,7.37 36.58,4.32 36.58,27.18 49.53,27.18 49.53,53.59 53.34,53.59

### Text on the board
tPlace: switchmodedesign.com
bPlace: L | S | L | S | L | S | L | S | L | S | L | S
tNames: N | P | N | P | N | P | N | N | N | P | N | N | N | P | N | N | N | P | N | N | GND | N | N | 170V | N

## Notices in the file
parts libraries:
SparkFun-Boards: Licensing: CC v3.0 Share-Alike You are welcome to use this library for commercial purposes.
